{attribute 'no-analysis'}
FUNCTION_BLOCK FB_Control EXTENDS FB_AsyncServiceResultClass IMPLEMENTS I_AcsiDataAccessEventClass, I_AcsiDataAccessCompletionClass
VAR
	_ipCtrl: I_AcsiCommonControllableDataClass; (* Interface pointer to controllable DO *)
	_eType: E_AcsiCDCType; (* CDC type of the controllable DO *)
	_ipBehVal: I_AcsiDATypeBeh; (* Interface pointer to value of 'Beh' DO of parent LN *)
	_ipStepSize: I_AcsiDATypeAnalogueValue; (* Interface pointer to DO containing stepsize information for BAC *)
	_ipCurrentAA: I_ScsmAssociationClass; (* Interface pointer to association for the current control procedure *)
	_stCurrrentIp: ST_SockAddr; (* IP address of the client for the current control procedure *)
	_ipLastApplErrorReq:  I_AsyncServiceResultClass; (*Interface pointer to LastApplError request service *)
	_nLastApplErrorReqState: BYTE; (* State of LastApplError transmission *)
	_ipCmdTermReq: I_AsyncServiceResultClass; (* Interface pointer to CommandTermination request service *)
	_nCmdTermReqState: BYTE; (* State of CommandTermination transmission *)
	bInit: BOOL; (* Indicates whether this function block has been initialized *)
	bNewState: BOOL; (* Indicates whether the ControlState changed in the last cycle *)
	bOperReq: BOOL; (* Indicates whether a valid Oper_req was received *)
	bSelReq: BOOL; (* Indicates whether a valid Sel_req was received *)
	bSelValReq: BOOL; (* Indicates whether a valid SelVal_req was received *)
	bCancelReq: BOOL; (* Indicates whether a valid Cancel_req was received *)
	fbCompletion: FB_AcsiServiceResultClass; (* Token for CompletionWaitEvent *)
	fbOperCompletion: FB_AcsiServiceResultClass; (* Token for CompletionWaitEvent of Oper_req *)
	fbSelValCompletion: FB_AcsiServiceResultClass; (* Token for CompletionWaitEvent of SelVal_req *)
	fbCancelCompletion: FB_AcsiServiceResultClass; (* Token for CompletionWaitEvent of Cancel_req *)
END_VAR

(* Checks if the value of 'Oper.ctlVal' is valid.
	Return value: TRUE => Value is valid; FALSE => Value is invalid. *)
METHOD PROTECTED _CheckCtlVal : BOOL
VAR_INPUT
	uCtlVal: U_AcsiCtlVal; (* Value of 'ctlVal' DA *)
END_VAR
VAR_OUTPUT
	eError: E_AcsiApplError; (* Error *)
	eAddCause: E_AcsiApplAddCause; (* Application error code *)
END_VAR
VAR
END_VAR
IF (_ipCtrl = 0) OR_ELSE (_eType = E_AcsiCDCType.none) THEN
	RETURN;
END_IF

CASE _eType OF
	E_AcsiCDCType.SPC:
		IF _ipCtrl.ipStVal_BOOLEAN = 0 THEN
			RETURN;
		END_IF
		IF uCtlVal.SPC = _ipCtrl.ipStVal_BOOLEAN.bValue THEN
			eError:= E_AcsiApplError.NoError;
			eAddCause:= E_AcsiApplAddCause.PositionReached;
		ELSE
			_CheckCtlVal:= TRUE;
		END_IF

	E_AcsiCDCType.DPC:
		IF _ipCtrl.ipStVal_Dbpos = 0 THEN
			RETURN;
		END_IF
		IF (SEL(uCtlVal.DPC, E_AcsiDbpos.Off, E_AcsiDbpos.On)) = _ipCtrl.ipStVal_Dbpos.eValue THEN
			eError:= E_AcsiApplError.NoError;
			eAddCause:= E_AcsiApplAddCause.PositionReached;
		ELSE
			_CheckCtlVal:= TRUE;
		END_IF

	E_AcsiCDCType.INC:
		IF _ipCtrl.ipStVal_INT32 = 0 THEN
			RETURN;
		END_IF
		IF uCtlVal.INC = _ipCtrl.ipStVal_INT32.iValue THEN
			eError:= E_AcsiApplError.NoError;
			eAddCause:= E_AcsiApplAddCause.PositionReached;
		ELSE
			_CheckCtlVal:= TRUE;
		END_IF

	E_AcsiCDCType.ENC:
		IF _ipCtrl.ipStVal_ENUMERATED = 0 THEN
			RETURN;
		END_IF
		IF uCtlVal.ENC.iAny = _ipCtrl.ipStVal_ENUMERATED.iAny THEN
			eError:= E_AcsiApplError.NoError;
			eAddCause:= E_AcsiApplAddCause.PositionReached;
		ELSE
			_CheckCtlVal:= TRUE;
		END_IF

	E_AcsiCDCType.BSC:
		IF _ipCtrl.ipValWTr = 0 THEN
			RETURN;
		END_IF
		CASE uCtlVal.BSC OF
			E_AcsiTcmd.Reserved:
				eError:= E_AcsiApplError.NoError;
				eAddCause:= E_AcsiApplAddCause.PositionReached;

			E_AcsiTcmd.Lower:
				IF _ipCtrl.ipValWTr.iPosVal = -64 THEN
					eError:= E_AcsiApplError.NoError;
					eAddCause:= E_AcsiApplAddCause.StepLimit;
				ELSE
					_CheckCtlVal:= TRUE;
				END_IF

			E_AcsiTcmd.Higher:
				IF _ipCtrl.ipValWTr.iPosVal = 63 THEN
					eError:= E_AcsiApplError.NoError;
					eAddCause:= E_AcsiApplAddCause.StepLimit;
				ELSE
					_CheckCtlVal:= TRUE;
				END_IF

			E_AcsiTcmd.Stop:
				_CheckCtlVal:= TRUE;
		END_CASE

	E_AcsiCDCType.ISC:
		IF _ipCtrl.ipValWTr = 0 THEN
			RETURN;
		END_IF
		IF (uCtlVal.ISC < -64) OR_ELSE (uCtlVal.ISC > 63) THEN
			eError:= E_AcsiApplError.NoError;
			eAddCause:= E_AcsiApplAddCause.InconsistentParameters;
		ELSE
			_CheckCtlVal:= TRUE;
		END_IF

	E_AcsiCDCType.APC:
		IF _ipCtrl.ipMxVal = 0 THEN
			RETURN;
		ELSE
			_CheckCtlVal:= TRUE;
		END_IF

	E_AcsiCDCType.BAC:
		IF _ipCtrl.ipMxVal = 0 THEN
			RETURN;
		ELSE
			CASE uCtlVal.BAC OF
				E_AcsiTcmd.Reserved:
					eError:= E_AcsiApplError.NoError;
					eAddCause:= E_AcsiApplAddCause.NotSupported;

				ELSE
					_CheckCtlVal:= TRUE;
			END_CASE
		END_IF
END_CASE
END_METHOD

(* Checks if the values of two 'ctlVal' are equal.
Return value: TRUE => Values are equal; FALSE => Values are unequal. *)
METHOD PROTECTED _CompareCtlVal : BOOL
VAR_INPUT
	uCtlVal1: U_AcsiCtlVal; (* Value of first 'ctlVal' *)
	uCtlVal2: U_AcsiCtlVal; (* Value of second 'ctlVal' *)
END_VAR
VAR
END_VAR
CASE _eType OF
	E_AcsiCDCType.SPC:
		_CompareCtlVal:= uCtlVal1.SPC = uCtlVal2.SPC;

	E_AcsiCDCType.DPC:
		_CompareCtlVal:= uCtlVal1.DPC = uCtlVal2.DPC;

	E_AcsiCDCType.INC:
		_CompareCtlVal:= uCtlVal1.INC = uCtlVal2.INC;

	E_AcsiCDCType.ENC:
		_CompareCtlVal:= uCtlVal1.ENC.iAny = uCtlVal2.ENC.iAny;

	E_AcsiCDCType.BSC:
		_CompareCtlVal:= uCtlVal1.BSC = uCtlVal2.BSC;

	E_AcsiCDCType.ISC:
		_CompareCtlVal:= uCtlVal1.ISC = uCtlVal2.ISC;

	E_AcsiCDCType.APC:
		_CompareCtlVal:= (uCtlVal1.APC.f = uCtlVal2.APC.f) AND_THEN (uCtlVal1.APC.i = uCtlVal2.APC.i);

	E_AcsiCDCType.BAC:
		_CompareCtlVal:= uCtlVal1.BAC = uCtlVal2.BAC;
END_CASE
END_METHOD

(* This method performs the operative test.
Since this test can take multiple PLC cycles, this method is called every cycle, until it returns TRUE. *)
METHOD PROTECTED _DynamicTest : BOOL
VAR_OUTPUT
	bDynamicTestOk: BOOL; (* Indicates whether the dynamic test was successful *)
	eError: E_AcsiServiceError; (* Error code for negative response *)
END_VAR
VAR
END_VAR
bDynamicTestOk:= TRUE;
_DynamicTest:= TRUE;
END_METHOD

(* Initializes the necessary local values. *)
METHOD PROTECTED _Init
VAR
END_VAR
IF _ipCtrl <> 0 THEN
	(* Set '_eType' according to CDC of the controllable data object *)
	IF _ipCtrl.sClass = 'SPC' THEN
		_eType:= E_AcsiCDCType.SPC;
	ELSIF _ipCtrl.sClass = 'DPC' THEN
		_eType:= E_AcsiCDCType.DPC;
	ELSIF _ipCtrl.sClass = 'INC' THEN
		_eType:= E_AcsiCDCType.INC;
	ELSIF _ipCtrl.sClass = 'ENC' THEN
		_eType:= E_AcsiCDCType.ENC;
	ELSIF _ipCtrl.sClass = 'BSC' THEN
		_eType:= E_AcsiCDCType.BSC;
	ELSIF _ipCtrl.sClass = 'ISC' THEN
		_eType:= E_AcsiCDCType.ISC;
	ELSIF _ipCtrl.sClass = 'APC' THEN
		_eType:= E_AcsiCDCType.APC;
	ELSIF _ipCtrl.sClass = 'BAC' THEN
		_eType:= E_AcsiCDCType.BAC;
	END_IF
	(* Get '_ipBehVal' *)
	IF _ipBehVal = 0 THEN
		_ipBehVal:= _ipCtrl.GetBehVal();
	END_IF
END_IF
END_METHOD

(* This method performs the operative test.
Since this test can take multiple PLC cycles, this method is called every cycle, until it returns TRUE. *)
METHOD PROTECTED _OperativeTest : BOOL
VAR_OUTPUT
	bOperativeTestOk: BOOL; (* Indicates whether the operative test was successful *)
	eError: E_AcsiServiceError; (* Error code for negative response *)
END_VAR
VAR
	eApplError: E_AcsiApplError;
	eApplAddCause: E_AcsiApplAddCause;
END_VAR
IF (_ipCtrl <> 0) AND_THEN (_ipCtrl.ipOper <> 0) THEN
	(* Don't allow Oper_req if 'ctlModel' is set to 'status-only' *)
	IF (_ipCtrl.ipCtlModel <> 0) AND_THEN (_ipCtrl.ipCtlModel.eValue = E_AcsiCtlModels.StatusOnly) THEN
		_SendLastApplError(ipAA:=_ipCurrentAA, ipCtrlData:=_ipCtrl.ipOper, eError:=E_AcsiApplError.NoError, ipOrigin:=_ipCtrl.ipOper.ipOrigin, ipCtlNum:=_ipCtrl.ipOper.ipCtlNum, eAddCause:=E_AcsiApplAddCause.Unknown);
		eError:= E_AcsiServiceError.AccessViolation;
		(* Check if Oper_req is valid for current value of 'Beh' *)
	ELSIF (_ipBehVal <> 0) AND_THEN ((_ipBehVal.eValue = E_AcsiBeh.Off) OR_ELSE ((_ipCtrl.ipOper.ipTest <> 0) AND_THEN (_ipCtrl.ipOper.ipTest.bValue <> ((_ipBehVal.eValue = E_AcsiBeh.Test) OR_ELSE (_ipBehVal.eValue = E_AcsiBeh.TestBlocked))))) THEN
		_SendLastApplError(ipAA:=_ipCurrentAA, ipCtrlData:=_ipCtrl.ipOper, eError:=E_AcsiApplError.NoError, ipOrigin:=_ipCtrl.ipOper.ipOrigin, ipCtlNum:=_ipCtrl.ipOper.ipCtlNum, eAddCause:=E_AcsiApplAddCause.BlockedByMode);
		eError:= E_AcsiServiceError.AccessViolation;
		(* Check if 'ctlVal' is valid *)
	ELSIF NOT _CheckCtlVal(uCtlVal:=_ipCtrl.ipOper.uCtlVal, eError=>eApplError, eAddCause=>eApplAddCause) THEN
		_SendLastApplError(ipAA:=_ipCurrentAA, ipCtrlData:=_ipCtrl.ipOper, eError:=eApplError, ipOrigin:=_ipCtrl.ipOper.ipOrigin, ipCtlNum:=_ipCtrl.ipOper.ipCtlNum, eAddCause:=eApplAddCause);
		eError:= E_AcsiServiceError.AccessViolation;
	ELSE (* Oper_req is valid *)
		RemoteAddress_From_ScsmAssociation(in:=_ipCurrentAA, out=>_stCurrrentIp);
		bOperativeTestOk:= TRUE;
	END_IF
END_IF
_OperativeTest:= TRUE;
END_METHOD

(* Resets all local values. *)
METHOD PROTECTED _Reset
VAR
END_VAR
(* Reset local values *)
_ipCurrentAA:= 0;
_stCurrrentIp.sAddr:= '';
_stCurrrentIp.nPort:= 0;
END_METHOD

(* Resets all values of the 'Cancel' DA to their configured initial values. *)
METHOD _ResetCancelValues
VAR
	ipCancel: I_AcsiDATypeCancel; (* Interface pointer to 'Cancel' DA *)
END_VAR
IF (_ipCtrl = 0) OR_ELSE ((ipCancel:=_ipCtrl.ipCancel) = 0) THEN
	RETURN;
END_IF

IF ipCancel.ipCtlVal <> 0 THEN
	ipCancel.uCtlVal:= ipCancel.uCtlVal_Config;
END_IF
IF ipCancel.ipOperTm <> 0 THEN
	ipCancel.ipOperTm.tValue:= ipCancel.ipOperTm.tConfig;
END_IF
IF ipCancel.ipOrigin <> 0 THEN
	ipCancel.ipOrigin.stOrigin:= ipCancel.ipOrigin.stConfig;
END_IF
IF ipCancel.ipCtlNum <> 0 THEN
	ipCancel.ipCtlNum.nValue:= ipCancel.ipCtlNum.nConfig;
END_IF
IF ipCancel.ipT <> 0 THEN
	ipCancel.ipT.tValue:= ipCancel.ipT.tConfig;
END_IF
IF ipCancel.ipTest <> 0 THEN
	ipCancel.ipTest.bValue:= ipCancel.ipTest.bConfig;
END_IF
END_METHOD

(* Resets all values of the 'Oper' DA to their configured initial values. *)
METHOD PROTECTED _ResetOperValues
VAR
	ipOper: I_AcsiDATypeOper; (* Interface pointer to 'Oper' DA *)
END_VAR
IF (_ipCtrl = 0) OR_ELSE ((ipOper:=_ipCtrl.ipOper) = 0) THEN
	RETURN;
END_IF

IF ipOper.ipCtlVal <> 0 THEN
	ipOper.uCtlVal:= ipOper.uCtlVal_Config;
END_IF
IF ipOper.ipOperTm <> 0 THEN
	ipOper.ipOperTm.tValue:= ipOper.ipOperTm.tConfig;
END_IF
IF ipOper.ipOrigin <> 0 THEN
	ipOper.ipOrigin.stOrigin:= ipOper.ipOrigin.stConfig;
END_IF
IF ipOper.ipCtlNum <> 0 THEN
	ipOper.ipCtlNum.nValue:= ipOper.ipCtlNum.nConfig;
END_IF
IF ipOper.ipT <> 0 THEN
	ipOper.ipT.tValue:= ipOper.ipT.tConfig;
END_IF
IF ipOper.ipTest <> 0 THEN
	ipOper.ipTest.bValue:= ipOper.ipTest.bConfig;
END_IF
END_METHOD

(* Resets all values of the 'SBOw' DA to their configured initial values. *)
METHOD PROTECTED _ResetSBOwValues
VAR
	ipSBOw: I_AcsiDATypeSBOw; (* Interface pointer to 'SBOw' DA *)
END_VAR
IF (_ipCtrl = 0) OR_ELSE ((ipSBOw:=_ipCtrl.ipSBOw) = 0) THEN
	RETURN;
END_IF

IF ipSBOw.ipCtlVal <> 0 THEN
	ipSBOw.uCtlVal:= ipSBOw.uCtlVal_Config;
END_IF
IF ipSBOw.ipOperTm <> 0 THEN
	ipSBOw.ipOperTm.tValue:= ipSBOw.ipOperTm.tConfig;
END_IF
IF ipSBOw.ipOrigin <> 0 THEN
	ipSBOw.ipOrigin.stOrigin:= ipSBOw.ipOrigin.stConfig;
END_IF
IF ipSBOw.ipCtlNum <> 0 THEN
	ipSBOw.ipCtlNum.nValue:= ipSBOw.ipCtlNum.nConfig;
END_IF
IF ipSBOw.ipT <> 0 THEN
	ipSBOw.ipT.tValue:= ipSBOw.ipT.tConfig;
END_IF
IF ipSBOw.ipTest <> 0 THEN
	ipSBOw.ipTest.bValue:= ipSBOw.ipTest.bConfig;
END_IF
IF ipSBOw.ipCheck <> 0 THEN
	ipSBOw.ipCheck.eValue:= ipSBOw.ipCheck.eConfig;
END_IF
END_METHOD

(* Sends a negative CommandTermination request. *)
METHOD PROTECTED _SendCommandTerminationReqNeg : BOOL
VAR_INPUT
	ipAA: I_ScsmAssociationClass; (* Interface pointer to application association *)
	ipCtrlData: I_AcsiCommonDataClass; (* Interface pointer to 'Oper', 'Cancel' or 'SBOw' control object, e.g. 'Relay1/XCBR1.CO.Pos.Oper', 'Relay1/CSWI1.CO.Pos.Cancel', 'Relay1/XCBR1.CO.Pos.SBOw' *)
	eError: E_AcsiApplError; (* Error *)
	ipOrigin: I_AcsiDATypeOriginator; (* Interface pointer to 'origin' attribute *)
	ipCtlNum: I_AcsiBATypeINT8U; (* Interface pointer to 'ctlNum' attribute *)
	eAddCause: E_AcsiApplAddCause; (* Application error code *)
END_VAR
VAR
	ipLastApplError: I_AcsiDATypeLastApplError;
END_VAR
IF (ipAA <> 0) AND_THEN (ipCtrlData <> 0) AND_THEN (ipOrigin <> 0) AND_THEN (ipCtlNum <> 0) THEN
	ipLastApplError:= ipAA.SetAdditionalCauseDiag(ipCtrlData:=_ipCtrl, eError:=eError, stOrigin:=ipOrigin.stOrigin, nCtlNum:=ipCtlNum.nValue, eAddCause:=eAddCause);
	ipAA.CommandTerminationReq(ipCtrlData:=ipCtrlData, ipLastApplError:=ipLastApplError, ipResult=>_ipCmdTermReq);
	_nCmdTermReqState:= 1;
END_IF
END_METHOD

(* Sends a positive CommandTermination request. *)
METHOD PROTECTED _SendCommandTerminationReqPos : BOOL
VAR_INPUT
	ipAA: I_ScsmAssociationClass; (* Interface pointer to application association *)
	ipCtrlData: I_AcsiCommonDataClass; (* Interface pointer to 'Oper', 'Cancel' or 'SBOw' control object, e.g. 'Relay1/XCBR1.CO.Pos.Oper', 'Relay1/CSWI1.CO.Pos.Cancel', 'Relay1/XCBR1.CO.Pos.SBOw' *)
END_VAR
VAR
END_VAR
IF (ipAA <> 0) AND_THEN (ipCtrlData <> 0) THEN
	_SendCommandTerminationReqPos:= ipAA.CommandTerminationReq(ipCtrlData:=ipCtrlData, ipLastApplError:=0, ipResult=>_ipCmdTermReq);
	_nCmdTermReqState:= 1;
END_IF
END_METHOD

(* Sends a LastApplError request. *)
METHOD PROTECTED _SendLastApplError : BOOL
VAR_INPUT
	ipAA: I_ScsmAssociationClass; (* Interface pointer to application association *)
	ipCtrlData: I_AcsiCommonDataClass; (* Interface pointer to 'Oper', 'Cancel' or 'SBOw' control object *)
	eError: E_AcsiApplError; (* Error *)
	ipOrigin: I_AcsiDATypeOriginator; (* Interface pointer to 'origin' attribute *)
	ipCtlNum: I_AcsiBATypeINT8U; (* Interface pointer to 'ctlNum' attribute *)
	eAddCause: E_AcsiApplAddCause; (* Application error code *)
END_VAR
VAR
	ipLastApplError: I_AcsiDATypeLastApplError; (* Interface pointer to AdditionalCauseDiag object *)
END_VAR
(* Get values from 'Oper' and send LastApplError *)
IF (ipAA <> 0) AND_THEN (ipOrigin <> 0) AND_THEN (ipCtlNum <> 0) THEN
	ipLastApplError:= ipAA.SetAdditionalCauseDiag(ipCtrlData:=ipCtrlData, eError:=eError, stOrigin:=ipOrigin.stOrigin, nCtlNum:=ipCtlNum.nValue, eAddCause:=eAddCause);

	_SendLastApplError:= ipAA.LastApplErrorReq(ipLastApplError:=ipLastApplError, ipResult=>_ipLastApplErrorReq);
	SUPER^.SetBusy();
	_nLastApplErrorReqState:= 1;
END_IF
END_METHOD

(* Sets the value of 'mxVal' to the value of 'ctlVal'.
Return value: TRUE => Success; FALSE => Failure. *)
METHOD PROTECTED _SetApcValue : BOOL
VAR_INPUT
	ipMxVal: I_AcsiDATypeAnalogueValue; (* Interface pointer to DA that will be written *)
	uCtlVal: U_AcsiCtlVal; (* Value of 'ctlVal' DA *)
	ipCtlVal_AV: I_AcsiDATypeAnalogueValue; (* Interface pointer to 'ctlVal' of type AnalogueValue *)
END_VAR
VAR
END_VAR
IF ((ipMxVal = 0) OR_ELSE ((ipMxVal.ipF = 0) AND_THEN (ipMxVal.ipI = 0))) OR_ELSE ((ipCtlVal_AV = 0) OR_ELSE ((ipCtlVal_AV.ipF = 0) AND_THEN (ipCtlVal_AV.ipI = 0))) THEN
	RETURN;
END_IF

IF ipMxVal.ipF <> 0 THEN
	IF ipCtlVal_AV.ipF <> 0 THEN
		ipMxVal.fValue:= uCtlVal.APC.f;
	ELSE
		(* 'ctlVal.i' is present, but not 'ctlVal.f' -> convert and use value of 'ctlVal.i' *)
		ipMxVal.fValue:= DINT_TO_REAL(uCtlVal.APC.i);
	END_IF
END_IF
IF ipMxVal.ipI <> 0 THEN
	IF ipCtlVal_AV.ipI <> 0 THEN
		ipMxVal.iValue:= uCtlVal.APC.i;
	ELSE
		(* 'ctlVal.if' is present, but not 'ctlVal.i' -> convert and use value of 'ctlVal.f' *)
		ipMxVal.iValue:= REAL_TO_DINT(uCtlVal.APC.f);
	END_IF
END_IF
END_METHOD

(* Increments or decrements the value of 'mxVal' according to the value of 'ctlVal' and 'stepSize'.
If 'stepSize' is not specified, the value 1 is used.
Return value: TRUE => Success; FALSE => Failure. *)
METHOD PROTECTED _SetBacValue : BOOL
VAR_INPUT
	ipMxVal: I_AcsiDATypeAnalogueValue; (* Interface pointer to DA that will be written *)
	uCtlVal: U_AcsiCtlVal; (* Value of 'ctlVal' DA *)
	ipStepSize: I_AcsiDATypeAnalogueValue; (* Interface pointer to 'stepSize' DA (Optional) *)
END_VAR
VAR
	fStepSize: REAL := 1; (* stepSize for 'f' *)
	iStepSize: DINT := 1; (* stepSize for 'i' *)
END_VAR
IF (ipMxVal = 0) OR_ELSE ((ipMxVal.ipF = 0) AND_THEN (ipMxVal.ipI = 0)) THEN
	RETURN;
END_IF

IF (ipStepSize <> 0) AND_THEN (((ipStepSize.ipF <> 0) AND_THEN (ipStepSize.fValue <> 0.0)) OR_ELSE ((ipStepSize.ipI <> 0) AND_THEN (ipStepSize.iValue <> 0))) THEN
	IF ipStepSize.ipF <> 0 THEN
		fStepSize:= ipStepSize.fValue;
	ELSE
		(* 'stepSize.i' is present, but not 'stepSize.f' -> convert and use value of 'stepSize.i' *)
		fStepSize:= DINT_TO_REAL(ipStepSize.iValue);
	END_IF
	IF ipStepSize.ipI <> 0 THEN
		iStepSize:= ipStepSize.iValue;
	ELSE
		(* 'stepSize.f' is present, but not 'stepSize.i' -> convert and use value of 'stepSize.f' *)
		iStepSize:= REAL_TO_DINT(ipStepSize.fValue);
	END_IF
END_IF

CASE uCtlVal.BAC OF
	E_AcsiTcmd.Stop:
		_SetBacValue:= TRUE;

	E_AcsiTcmd.Lower:
		IF ipMxVal.ipF <> 0 THEN
			ipMxVal.fValue:= ipMxVal.fValue - fStepSize;
		END_IF
		IF ipMxVal.ipI <> 0 THEN
			ipMxVal.iValue:= ipMxVal.iValue - iStepSize;
		END_IF
		_SetBacValue:= TRUE;

	E_AcsiTcmd.Higher:
		IF ipMxVal.ipF <> 0 THEN
			ipMxVal.fValue:= ipMxVal.fValue + fStepSize;
		END_IF
		IF ipMxVal.ipI <> 0 THEN
			ipMxVal.iValue:= ipMxVal.iValue + iStepSize;
		END_IF
		_SetBacValue:= TRUE;
END_CASE
END_METHOD

(* Increments or decrements the value of 'valWTr' according to the value of 'ctlVal'.
Return value: TRUE => Success; FALSE => Failure. *)
METHOD PROTECTED _SetBscValue : BOOL
VAR_INPUT
	ipValWTr: I_AcsiDATypeValWithTrans; (* Interface pointer to DA that will be written *)
	uCtlVal: U_AcsiCtlVal; (* Value of 'ctlVal' DA *)
END_VAR
VAR
END_VAR
IF ipValWTr = 0 THEN
	RETURN;
END_IF

CASE uCtlVal.BSC OF
	E_AcsiTcmd.Stop:
		_SetBscValue:= TRUE;

	E_AcsiTcmd.Lower:
		ipValWTr.iPosVal:= ipValWTr.iPosVal - 1;
		_SetBscValue:= TRUE;

	E_AcsiTcmd.Higher:
		ipValWTr.iPosVal:= ipValWTr.iPosVal + 1;
		_SetBscValue:= TRUE;
END_CASE
END_METHOD

(* Sets the value of 'stVal' according to the value of 'ctlVal'.
Return value: TRUE => Success; FALSE => Failure. *)
METHOD PROTECTED _SetDpcValue : BOOL
VAR_INPUT
	ipStVal: I_AcsiDATypeDbpos; (* Interface pointer to DA that will be written *)
	uCtlVal: U_AcsiCtlVal; (* Value of 'ctlVal' DA *)
END_VAR
VAR
END_VAR
IF ipStVal = 0 THEN
	RETURN;
END_IF

ipStVal.eValue:= SEL(uCtlVal.DPC, E_AcsiDbpos.Off, E_AcsiDbpos.On);
_SetDpcValue:= TRUE;
END_METHOD

(* Sets the value of 'stVal' according to the value of 'ctlVal'.
Return value: TRUE => Success; FALSE => Failure. *)
METHOD PROTECTED _SetEncValue : BOOL
VAR_INPUT
	ipStVal: I_AcsiBATypeENUMERATED; (* Interface pointer to DA that will be written *)
	uCtlVal: U_AcsiCtlVal; (* Value of 'ctlVal' DA *)
END_VAR
VAR
END_VAR
IF ipStVal = 0 THEN
	RETURN;
END_IF

ipStVal.iAny:= uCtlVal.ENC.iAny;
_SetEncValue:= TRUE;
END_METHOD

(* Sets the value of 'stVal' to the value of 'ctlVal'.
Return value: TRUE => Success; FALSE => Failure. *)
METHOD PROTECTED _SetIncValue : BOOL
VAR_INPUT
	ipStVal: I_AcsiBATypeINT32; (* Interface pointer to DA that will be written *)
	uCtlVal: U_AcsiCtlVal; (* Value of 'ctlVal' DA *)
END_VAR
VAR
END_VAR
IF ipStVal = 0 THEN
	RETURN;
END_IF

ipStVal.iValue:= uCtlVal.INC;
_SetIncValue:= TRUE;
END_METHOD

(* Sets the value of 'valWTr' to the value of 'ctlVal'.
Return value: TRUE => Success; FALSE => Failure. *)
METHOD PROTECTED _SetIscValue : BOOL
VAR_INPUT
	ipValWTr: I_AcsiDATypeValWithTrans; (* Interface pointer to DA that will be written *)
	uCtlVal: U_AcsiCtlVal; (* Value of 'ctlVal' DA *)
END_VAR
VAR
END_VAR
IF ipValWTr = 0 THEN
	RETURN;
END_IF

ipValWTr.iPosVal:= uCtlVal.ISC;
_SetIscValue:= TRUE;
END_METHOD

(* Sets the value of 'stVal' to the value of 'ctlVal'.
Return value: TRUE => Success; FALSE => Failure. *)
METHOD PROTECTED _SetSpcValue : BOOL
VAR_INPUT
	ipStVal: I_AcsiBATypeBOOLEAN; (* Interface pointer to DA that will be written *)
	uCtlVal: U_AcsiCtlVal; (* Value of 'ctlVal' DA *)
END_VAR
VAR
END_VAR
IF ipStVal = 0 THEN
	RETURN;
END_IF

ipStVal.bValue:= uCtlVal.SPC;
_SetSpcValue:= TRUE;
END_METHOD

(* Sets the value of the respective DA according to the value of 'Oper.ctlVal'.
Return value: TRUE => Success, FALSE => Failure. *)
METHOD PROTECTED _SetValue : BOOL
VAR_INPUT
	uCtlVal: U_AcsiCtlVal; (* Value of 'ctlVal' DA *)
	ipCtlVal_AV: I_AcsiDATypeAnalogueValue; (* Interface pointer to 'ctlVal' of type AnalogueValue *)
END_VAR
VAR
END_VAR
IF _ipCtrl = 0 THEN
	RETURN;
END_IF

CASE _eType OF
	E_AcsiCDCType.SPC:
		_SetValue:= _SetSpcValue(ipStVal:=_ipCtrl.ipStVal_BOOLEAN, uCtlVal:=uCtlVal);

	E_AcsiCDCType.DPC:
		_SetValue:= _SetDpcValue(ipStVal:=_ipCtrl.ipStVal_Dbpos, uCtlVal:=uCtlVal);

	E_AcsiCDCType.INC:
		_SetValue:= _SetIncValue(ipStVal:=_ipCtrl.ipStVal_INT32, uCtlVal:=uCtlVal);

	E_AcsiCDCType.ENC:
		_SetValue:= _SetEncValue(ipStVal:=_ipCtrl.ipStVal_ENUMERATED, uCtlVal:=uCtlVal);

	E_AcsiCDCType.BSC:
		_SetValue:= _SetBscValue(ipValWTr:=_ipCtrl.ipValWTr, uCtlVal:=uCtlVal);

	E_AcsiCDCType.ISC:
		_SetValue:= _SetIscValue(ipValWTr:=_ipCtrl.ipValWTr, uCtlVal:=uCtlVal);

	E_AcsiCDCType.APC:
		_SetValue:= _SetApcValue(ipMxVal:=_ipCtrl.ipMxVal, uCtlVal:=uCtlVal, ipCtlVal_AV:=ipCtlVal_AV);

	E_AcsiCDCType.BAC:
		_SetValue:= _SetBacValue(ipMxVal:=_ipCtrl.ipMxVal, uCtlVal:=uCtlVal, ipStepSize:=_ipStepSize);

END_CASE
END_METHOD

(* This method performs the test of the SelectWithValue operation.
Since this test can take multiple PLC cycles, this method is called every cycle, until it returns TRUE. *)
METHOD PROTECTED _Test : BOOL
VAR_OUTPUT
	bTestOk: BOOL; (* Indicates whether the test was successful *)
	eError: E_AcsiServiceError; (* Error code for negative response *)
END_VAR
VAR
	eApplError: E_AcsiApplError; (* Error *)
	eApplAddCause: E_AcsiApplAddCause; (* Application error code *)
END_VAR
IF (_ipCtrl <> 0) AND_THEN (_ipCtrl.ipSBOw <> 0) THEN
	(* Don't allow control if 'ctlModel' is set to 'status-only' *)
	IF (_ipCtrl.ipCtlModel <> 0) AND_THEN (_ipCtrl.ipCtlModel.eValue = E_AcsiCtlModels.StatusOnly) THEN
		_SendLastApplError(ipAA:=_ipCurrentAA, ipCtrlData:=_ipCtrl.ipSBOw, eError:=E_AcsiApplError.NoError, ipOrigin:=_ipCtrl.ipSBOw.ipOrigin, ipCtlNum:=_ipCtrl.ipSBOw.ipCtlNum, eAddCause:=E_AcsiApplAddCause.Unknown);
		eError:= E_AcsiServiceError.AccessViolation;
		(* Check if 'ctlVal' is valid *)
	ELSIF NOT _CheckCtlVal(uCtlVal:=_ipCtrl.ipSBOw.uCtlVal, eError=>eApplError, eAddCause=>eApplAddCause) THEN
		_SendLastApplError(ipAA:=_ipCurrentAA, ipCtrlData:=_ipCtrl.ipSBOw, eError:=eApplError, ipOrigin:=_ipCtrl.ipSBOw.ipOrigin, ipCtlNum:=_ipCtrl.ipSBOw.ipCtlNum, eAddCause:=eApplAddCause);
		eError:= E_AcsiServiceError.AccessViolation;
		(* SelVal_req is valid *)
	ELSE
		RemoteAddress_From_ScsmAssociation(in:=_ipCurrentAA, out=>_stCurrrentIp);
		bTestOk:= TRUE;
	END_IF
END_IF
_Test:= TRUE;
END_METHOD

(* Sets the value of 't' to the current time.
Return value: TRUE => Success; FALSE => Failure. *)
METHOD PROTECTED _UpdateTimestampValue : BOOL
VAR_INPUT
	ipAA: I_ScsmAssociationClass; (* Interface pointer to application association *)
END_VAR
VAR
	tValue: T_UtcTime; (* Current time *)
END_VAR
IF (ipAA <> 0) AND_THEN (_ipCtrl <> 0) AND_THEN (_ipCtrl.ipT <> 0) THEN
	_UpdateTimestampValue:= ipAA.GetSystemTime(tT=>tValue);
	_ipCtrl.ipT.tValue:= tValue;
END_IF
END_METHOD

PROPERTY eType : E_AcsiCDCType
GET
eType:= _eType;
END_GET
SET
_eType:= eType;
END_SET
END_PROPERTY

PROPERTY ipBehVal : I_AcsiDATypeBeh
GET
ipBehVal:= _ipBehVal;
END_GET
SET
_ipBehVal:= ipBehVal;
END_SET
END_PROPERTY

PROPERTY ipCtrl : I_AcsiCommonControllableDataClass
GET
ipCtrl:= _ipCtrl;
END_GET
SET
_ipCtrl:= ipCtrl;
END_SET
END_PROPERTY

PROPERTY ipStepSize : I_AcsiDATypeAnalogueValue
GET
ipStepSize:= _ipStepSize;
END_GET
SET
_ipStepSize:= ipStepSize;
END_SET
END_PROPERTY

METHOD OnAbort : BOOL
VAR_INPUT
	ipReason: I_ServiceErrorClass;
END_VAR
VAR_OUTPUT
	ipResult: I_AsyncServiceResultClass := THIS^;
END_VAR
VAR
END_VAR
(* Forward Abort to LastApplError request service *)
IF (_ipLastApplErrorReq <> 0) AND_THEN (_ipLastApplErrorReq.IsBusy()) THEN
	_ipLastApplErrorReq.OnAbort(ipReason:=ipReason);
END_IF
(* Forward Abort to CommandTermination request service *)
IF (_ipCmdTermReq <> 0) AND_THEN (_ipCmdTermReq.IsBusy()) THEN
	_ipCmdTermReq.OnAbort(ipReason:=ipReason);
END_IF

SUPER^.SetCompleted();
fbCompletion.SetCompleted();
END_METHOD

METHOD OnCompletionWaitEvent : BOOL
VAR_INPUT
	ipDai: I_AcsiDataAccessInfoClass;
	ipData: I_AcsiCommonDataClass;
	eFc: E_AcsiFc;
END_VAR
VAR_OUTPUT
	ipResult: I_AcsiServiceResultClass := fbCompletion;
END_VAR
VAR
END_VAR
END_METHOD

(* Implementation of user application data update event method. *)
METHOD OnGetVEvent
VAR_INPUT
	ipDai: I_AcsiDataAccessInfoClass; (* Additional data access info *)
	ipData: I_AcsiCommonDataClass; (* Interface pointer to data object *)
	eFc: E_AcsiFc; (* Functional constraint *)
END_VAR
VAR
END_VAR
END_METHOD

(* Implementation of user application data update event method. *)
METHOD OnGetVPreEvent : E_AcsiServiceError
VAR_INPUT
	ipDai: I_AcsiDataAccessInfoClass; (* Additional data access info *)
	ipData: I_AcsiCommonDataClass; (* Interface pointer to data object *)
	eFc: E_AcsiFc; (* Functional constraint *)
END_VAR
VAR
END_VAR
END_METHOD

(* Implementation of user application data update event method. *)
METHOD OnSetVEvent
VAR_INPUT
	ipDai: I_AcsiDataAccessInfoClass; (* Additional data access info *)
	ipData: I_AcsiCommonDataClass; (* Interface pointer to data object *)
	eFc: E_AcsiFc; (* Functional constraint *)
END_VAR
VAR
END_VAR
END_METHOD

(* Implementation of user application data update event method. *)
METHOD OnSetVPreEvent : E_AcsiServiceError
VAR_INPUT
	ipDai: I_AcsiDataAccessInfoClass; (* Additional data access info *)
	ipMemory: I_AnyMemoryBuffer; (* Interface pointer to buffer containig new value data *)
	ipData: I_AcsiCommonDataClass; (* Interface pointer to data object *)
	eFc: E_AcsiFc; (* Functional constraint *)
END_VAR
VAR_OUTPUT
	ipLastApplError: I_AcsiDATypeLastApplError; (* IF <> 0 => send LastApplError request *)
END_VAR
VAR
END_VAR
END_METHOD

END_FUNCTION_BLOCK
